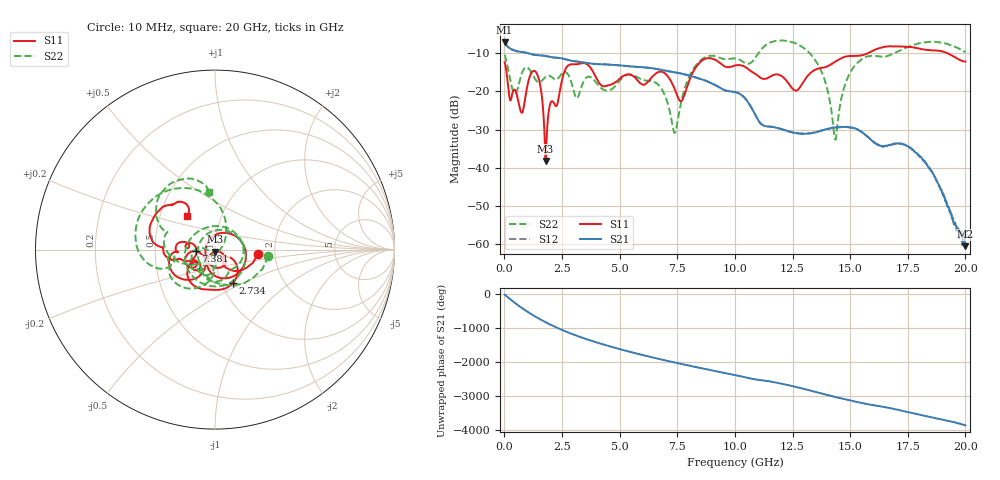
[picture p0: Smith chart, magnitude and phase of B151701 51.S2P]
!  2-Port S-parameters saved by WinCal
! VAR MeasName=S-Parameters (CALIBRATED_DATA) read from VNA (N5244A)
! VAR MeasDate=2015-12-24 19:15:32
! VAR NAME=B151701 51
! VAR FILENAME=B151701 51.S2P
! VAR DATE=2015-12-24 19:15:32
! VAR PHYS_PORTS=1,3
# Hz S DB R 50
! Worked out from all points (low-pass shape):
!   801 points, 10 MHz to 20 GHz, reference 50 ohm
!   highest |S21| = -7.17 dB at 10 MHz (marker M1); lowest = -60.5 dB at 20 GHz (marker M2)
!   |S21| within 3 dB of the highest: start of sweep to 1.077 GHz
!   lowest |S11| = -38.2 dB at 1.784 GHz (marker M3), VSWR 1.02, Z = 50 - j1.23 ohm
!   |S11| at or under -10 dB: start of sweep to 15.8 GHz; 19.18 GHz to end of sweep
!   |S22| runs from -32.6 to -6.7 dB; largest |S21 - S12| = 0.001
!   S11 on the Smith chart (normalised r, x): 10 MHz: 1.62, -0.08; 2.734 GHz: 1.13, -0.44; 7.381 GHz: 0.81, -0.02; 20 GHz: 0.69, +0.27
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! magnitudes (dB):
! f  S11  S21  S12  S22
! 10 MHz  -12.4  -7.2  -7.1  -10.5
! 409.8 MHz  -19.6  -9.3  -9.3  -20.4
! 734.6 MHz  -25.5  -9.7  -9.7  -15.8
! 1.384 GHz  -15.1  -10.5  -10.5  -17.3
! 1.784 GHz  -38.2  -10.8  -10.8  -16.3
! 2.734 GHz  -13.5  -11.8  -11.8  -15.4
! 3.108 GHz  -13.0  -12.2  -12.2  -21.7
! 3.358 GHz  -12.7  -12.4  -12.4  -18.6
! 4.308 GHz  -18.7  -13.0  -13.0  -19.6
! 6.682 GHz  -15.0  -14.3  -14.3  -18.3
! 7.381 GHz  -19.4  -15.1  -15.0  -30.9
! 7.706 GHz  -22.4  -15.4  -15.5  -21.9
! 8.381 GHz  -13.1  -16.5  -16.6  -12.7
! 10.01 GHz  -13.3  -20.2  -20.2  -11.4
! 12.63 GHz  -19.8  -30.9  -30.9  -7.5
! 13.35 GHz  -14.9  -30.9  -30.9  -10.8
! 13.93 GHz  -13.7  -29.9  -30.0  -17.8
! 14.35 GHz  -12.3  -29.5  -29.5  -32.6
! 15.13 GHz  -10.8  -29.6  -29.7  -13.9
! 16.68 GHz  -8.3  -34.0  -34.1  -10.7
! 18.18 GHz  -9.1  -38.1  -38.1  -7.3
! 20 GHz  -12.3  -60.5  -59.0  -9.8
